| Teraspeed Modeling Services.
| http://www.teraspeedlabs.com
[IBIS Ver]   4.0
[Comment Char] |_char
[File Name]   lpc54113j256uk49.ibs
[File Rev]   3.0
[Source]  Measured and created by Teraspeed Labs
[Date]   10-25-2017
[Notes]   Quality Check of this IBIS model: Model Passes IBIS Check
   Model parses into ICX IS. Simulation done with Hyperlynx.
   1. MIN TYP MAX information is based on Temperature and Voltage
   characteristics only.
   2. Package data measured using Tektronix IConnect Software.
[Disclaimer]
| Use: Teraspeed Labs ("Teraspeed") has
| licensed IBIS models to specific integrated circuit
| suppliers ("IC Vendors") for use and distribution as
| follows: Each IC Vendor may use IBIS Models, and distribute
| them to IC Vendor's customers to use solely for developing
| printed circuit board designs. Users of this model may
| modify the IBIS model to suit its specific applications but
| rights to derivative works and such modifications shall belong
| to Teraspeed. No other distribution of these materials is
| permitted.
| DISCLAIMER OF WARRANTY: UNLESS OTHERWISE AGREED TO IN WRITING
| TERASPEED DISCLAIMS AND USER WAIVES ALL WARRANTIES, EXPRESS
| OR IMPLIED, INCLUDING WARRANTIES OF MERCHANTABILITY AND
| FITNESS FOR A PARTICULAR PURPOSE. IN NO EVENT SHALL
| TERASPEED BE LIABLE FOR ANY DIRECT OR INDIRECT DAMAGES,
| WHETHER IN CONTRACT OR TORT, INCLUDING, WITHOUT LIMITATION,
| LOST PROFITS, BUSINESS INTERRUPTION, OR LOST INFORMATION
| ARISING OUT OF THE USE OF OR THE INABILITY TO USE THE MODEL,
| EVEN IF TERASPEED HAS BEEN ADVISED OF THE POSSIBILITY OF SUCH
| DAMAGES.
[Copyright]
| This file is the legal property of Teraspeed Labs Copyright(c) 2017.
| All other rights are reserved.
[Component] LPC54113J256UK49
[Manufacturer] NXP Semiconductors
| Data Sheet: Rev 1.2, 24 February 2016
[Package]
| 49 Ball BGA / WLCSP49
| variable   typ   min   max
R_pkg  1.000E-02  1.000E-02  1.000E-02
L_pkg  5.322E-10  1.768E-10  7.500E-10
C_pkg  2.129E-14  7.071E-15  3.000E-14
[Pin] signal_name  model_name  R_pin  L_pin C_pin
A1   PIO1_2/ADC0_5   pio1_2   1.000E-02   7.500E-10   3.000E-14
A2   PIO1_4/ADC0_7   pio1_4   1.000E-02   6.374E-10   2.550E-14
A3   VSSA   GND   1.000E-02   7.500E-10   3.000E-14
A4   VDDA   POWER   1.000E-02   7.500E-10   3.000E-14
A5   PIO1_6/ADC0_9   pio1_6   1.000E-02   5.590E-10   2.236E-14
A6   PIO0_0   pio0_0   1.000E-02   6.374E-10   2.550E-14
A7   RTCXIN   rtcxin   1.000E-02   7.500E-10   3.000E-14
B1   PIO1_1/ADC0_4   pio1_1   1.000E-02   6.374E-10   2.550E-14
B2   PIO1_3/ADC0_6   pio1_3   1.000E-02   5.000E-10   2.000E-14
B3   PIO1_5/ADC0_8   pio1_5   1.000E-02   3.953E-10   1.581E-14
B4   VREFP   POWER   1.000E-02   7.500E-10   3.000E-14
B5   PIO1_7/ADC0_10   pio1_7   1.000E-02   3.953E-10   1.581E-14
B6   PIO0_1   pio0_1   1.000E-02   5.000E-10   2.000E-14
B7   RTCXOUT   rtcxout   1.000E-02   6.374E-10   2.550E-14
C1   PIO0_30/ADC0_1   pio0_30   1.000E-02   5.590E-10   2.236E-14
C2   PIO0_31/ADC0_2   pio0_31   1.000E-02   3.953E-10   1.581E-14
C3   PIO1_0/ADC0_3   pio1_0   1.000E-02   2.500E-10   1.000E-14
C4   VDD   POWER   1.000E-02   7.500E-10   3.000E-14
C5   PIO1_8/ADC0_11   pio1_8   1.000E-02   2.500E-10   1.000E-14
C6   PIO0_5   pio0_5   1.000E-02   3.953E-10   1.581E-14
C7   PIO0_4   pio0_4   1.000E-02   5.590E-10   2.236E-14
D1   USB_DM   analog_io   1.000E-02   5.303E-10   2.121E-14
D2   USB_DP   analog_io   1.000E-02   3.536E-10   1.414E-14
D3   PIO0_29/ADC0_0   pio0_29   1.000E-02   1.768E-10   7.071E-15
D4   VSS   GND   1.000E-02   7.500E-10   3.000E-14
D5   PIO0_8   pio0_8   1.000E-02   1.768E-10   7.071E-15
D6   PIO0_7   pio0_7   1.000E-02   3.536E-10   1.414E-14
D7   PIO0_6   pio0_6   1.000E-02   5.303E-10   2.121E-14
E1   PIO0_26   pio0_26   1.000E-02   5.590E-10   2.236E-14
E2   PIO0_25   pio0_25   1.000E-02   3.953E-10   1.581E-14
E3   PIO0_21   pio0_21   1.000E-02   2.500E-10   1.000E-14
E4   VSS   GND   1.000E-02   7.500E-10   3.000E-14
E5   PIO0_11   pio0_11   1.000E-02   2.500E-10   1.000E-14
E6   PIO0_10   pio0_10   1.000E-02   3.953E-10   1.581E-14
E7   PIO0_9   pio0_9   1.000E-02   5.590E-10   2.236E-14
F1   PIO0_24   pio0_24   1.000E-02   6.374E-10   2.550E-14
F2   PIO0_23   pio0_23   1.000E-02   5.000E-10   2.000E-14
F3   PIO0_20/TMS   pio0_20   1.000E-02   3.953E-10   1.581E-14
F4   VDD   POWER   1.000E-02   7.500E-10   3.000E-14
F5   SWCLK/PIO0_16   pio0_16   1.000E-02   3.953E-10   1.581E-14
F6   PIO0_14/TCK   pio0_14   1.000E-02   5.000E-10   2.000E-14
F7   PIO0_12   pio0_12   1.000E-02   6.374E-10   2.550E-14
G1   *RESET   reset   1.000E-02   7.500E-10   3.000E-14
G2   PIO0_22   pio0_22   1.000E-02   6.374E-10   2.550E-14
G3   PIO0_19/TDI   pio0_19   1.000E-02   5.590E-10   2.236E-14
G4   PIO0_18/*TRST   pio0_18   1.000E-02   5.303E-10   2.121E-14
G5   SWDIO/PIO0_17   pio0_17   1.000E-02   5.590E-10   2.236E-14
G6   PIO0_15/TDO   pio0_15   1.000E-02   6.374E-10   2.550E-14
G7   PIO0_13   pio0_13   1.000E-02   7.500E-10   3.000E-14
|**Open drain io pins
[Model Selector]   pio0_23
i2c_norm_hi_1.8v   i2c norm mode,hi drv,Open Drain io,1.8V
i2c_norm_hi_2.5v   i2c norm mode,hi drv,Open Drain io,2.5V
i2c_norm_hi_3.3v   i2c norm mode,hi drv,Open Drain io,3.3V
i2c_norm_lo_1.8v   i2c norm mode,lo drv,Open Drain io,1.8V
i2c_norm_lo_2.5v   i2c norm mode,lo drv,Open Drain io,2.5V
i2c_norm_lo_3.3v   i2c norm mode,lo drv,Open Drain io,3.3V
[Model Selector]   pio0_24
i2c_norm_hi_1.8v   i2c norm mode,hi drv,Open Drain io,1.8V
i2c_norm_hi_2.5v   i2c norm mode,hi drv,Open Drain io,2.5V
i2c_norm_hi_3.3v   i2c norm mode,hi drv,Open Drain io,3.3V
i2c_norm_lo_1.8v   i2c norm mode,lo drv,Open Drain io,1.8V
i2c_norm_lo_2.5v   i2c norm mode,lo drv,Open Drain io,2.5V
i2c_norm_lo_3.3v   i2c norm mode,lo drv,Open Drain io,3.3V
[Model Selector]   pio0_25
i2c_norm_hi_1.8v   i2c norm mode,hi drv,Open Drain io,1.8V
i2c_norm_hi_2.5v   i2c norm mode,hi drv,Open Drain io,2.5V
i2c_norm_hi_3.3v   i2c norm mode,hi drv,Open Drain io,3.3V
i2c_norm_lo_1.8v   i2c norm mode,lo drv,Open Drain io,1.8V
i2c_norm_lo_2.5v   i2c norm mode,lo drv,Open Drain io,2.5V
i2c_norm_lo_3.3v   i2c norm mode,lo drv,Open Drain io,3.3V
[Model Selector]   pio0_26
i2c_norm_hi_1.8v   i2c norm mode,hi drv,Open Drain io,1.8V
i2c_norm_hi_2.5v   i2c norm mode,hi drv,Open Drain io,2.5V
i2c_norm_hi_3.3v   i2c norm mode,hi drv,Open Drain io,3.3V
i2c_norm_lo_1.8v   i2c norm mode,lo drv,Open Drain io,1.8V
i2c_norm_lo_2.5v   i2c norm mode,lo drv,Open Drain io,2.5V
i2c_norm_lo_3.3v   i2c norm mode,lo drv,Open Drain io,3.3V
|**Standard io pins,5Vtol
[Model Selector]   pio0_0
pio_1.8v   GP io,1.8V
pio_2.5v   GP io,2.5V
pio_3.3v   GP io,3.3V
pio_1.8v_pd   GP io,pd,1.8V
pio_2.5v_pd   GP io,pd,2.5V
pio_3.3v_pd   GP io,pd,3.3V
pio_1.8v_pu   GP io,pu,1.8V | Pwrup Default
pio_2.5v_pu   GP io,pu,2.5V | Pwrup Default
pio_3.3v_pu   GP io,pu,3.3V | Pwrup Default
pio_fast_1.8v   GP io,fast slew,1.8V
pio_fast_2.5v   GP io,fast slew,2.5V
pio_fast_3.3v   GP io,fast slew,3.3V
pio_fast_1.8v_pd   GP io,fast slew,pd,1.8V
pio_fast_2.5v_pd   GP io,fast slew,pd,2.5V
pio_fast_3.3v_pd   GP io,fast slew,pd,3.3V
pio_fast_1.8v_pu   GP io,fast slew,pu,1.8V
pio_fast_2.5v_pu   GP io,fast slew,pu,2.5V
pio_fast_3.3v_pu   GP io,fast slew,pu,3.3V
[Model Selector]   pio0_1
pio_1.8v   GP io,1.8V
pio_2.5v   GP io,2.5V
pio_3.3v   GP io,3.3V
pio_1.8v_pd   GP io,pd,1.8V
pio_2.5v_pd   GP io,pd,2.5V
pio_3.3v_pd   GP io,pd,3.3V
pio_1.8v_pu   GP io,pu,1.8V | Pwrup Default
pio_2.5v_pu   GP io,pu,2.5V | Pwrup Default
pio_3.3v_pu   GP io,pu,3.3V | Pwrup Default
pio_fast_1.8v   GP io,fast slew,1.8V
pio_fast_2.5v   GP io,fast slew,2.5V
pio_fast_3.3v   GP io,fast slew,3.3V
pio_fast_1.8v_pd   GP io,fast slew,pd,1.8V
pio_fast_2.5v_pd   GP io,fast slew,pd,2.5V
pio_fast_3.3v_pd   GP io,fast slew,pd,3.3V
pio_fast_1.8v_pu   GP io,fast slew,pu,1.8V
pio_fast_2.5v_pu   GP io,fast slew,pu,2.5V
pio_fast_3.3v_pu   GP io,fast slew,pu,3.3V
[Model Selector]   pio0_4
pio_1.8v   GP io,1.8V
pio_2.5v   GP io,2.5V
pio_3.3v   GP io,3.3V
pio_1.8v_pd   GP io,pd,1.8V
pio_2.5v_pd   GP io,pd,2.5V
pio_3.3v_pd   GP io,pd,3.3V
pio_1.8v_pu   GP io,pu,1.8V | Pwrup Default
pio_2.5v_pu   GP io,pu,2.5V | Pwrup Default
pio_3.3v_pu   GP io,pu,3.3V | Pwrup Default
pio_fast_1.8v   GP io,fast slew,1.8V
pio_fast_2.5v   GP io,fast slew,2.5V
pio_fast_3.3v   GP io,fast slew,3.3V
pio_fast_1.8v_pd   GP io,fast slew,pd,1.8V
pio_fast_2.5v_pd   GP io,fast slew,pd,2.5V
pio_fast_3.3v_pd   GP io,fast slew,pd,3.3V
pio_fast_1.8v_pu   GP io,fast slew,pu,1.8V
pio_fast_2.5v_pu   GP io,fast slew,pu,2.5V
pio_fast_3.3v_pu   GP io,fast slew,pu,3.3V
[Model Selector]   pio0_5
pio_1.8v   GP io,1.8V
pio_2.5v   GP io,2.5V
pio_3.3v   GP io,3.3V
pio_1.8v_pd   GP io,pd,1.8V
pio_2.5v_pd   GP io,pd,2.5V
pio_3.3v_pd   GP io,pd,3.3V
pio_1.8v_pu   GP io,pu,1.8V | Pwrup Default
pio_2.5v_pu   GP io,pu,2.5V | Pwrup Default
pio_3.3v_pu   GP io,pu,3.3V | Pwrup Default
pio_fast_1.8v   GP io,fast slew,1.8V
pio_fast_2.5v   GP io,fast slew,2.5V
pio_fast_3.3v   GP io,fast slew,3.3V
pio_fast_1.8v_pd   GP io,fast slew,pd,1.8V
pio_fast_2.5v_pd   GP io,fast slew,pd,2.5V
pio_fast_3.3v_pd   GP io,fast slew,pd,3.3V
pio_fast_1.8v_pu   GP io,fast slew,pu,1.8V
pio_fast_2.5v_pu   GP io,fast slew,pu,2.5V
pio_fast_3.3v_pu   GP io,fast slew,pu,3.3V
[Model Selector]   pio0_6
pio_1.8v   GP io,1.8V
pio_2.5v   GP io,2.5V
pio_3.3v   GP io,3.3V
pio_1.8v_pd   GP io,pd,1.8V
pio_2.5v_pd   GP io,pd,2.5V
pio_3.3v_pd   GP io,pd,3.3V
pio_1.8v_pu   GP io,pu,1.8V | Pwrup Default
pio_2.5v_pu   GP io,pu,2.5V | Pwrup Default
pio_3.3v_pu   GP io,pu,3.3V | Pwrup Default
pio_fast_1.8v   GP io,fast slew,1.8V
pio_fast_2.5v   GP io,fast slew,2.5V
pio_fast_3.3v   GP io,fast slew,3.3V
pio_fast_1.8v_pd   GP io,fast slew,pd,1.8V
pio_fast_2.5v_pd   GP io,fast slew,pd,2.5V
pio_fast_3.3v_pd   GP io,fast slew,pd,3.3V
pio_fast_1.8v_pu   GP io,fast slew,pu,1.8V
pio_fast_2.5v_pu   GP io,fast slew,pu,2.5V
pio_fast_3.3v_pu   GP io,fast slew,pu,3.3V
[Model Selector]   pio0_7
pio_1.8v   GP io,1.8V
pio_2.5v   GP io,2.5V
pio_3.3v   GP io,3.3V
pio_1.8v_pd   GP io,pd,1.8V
pio_2.5v_pd   GP io,pd,2.5V
pio_3.3v_pd   GP io,pd,3.3V
pio_1.8v_pu   GP io,pu,1.8V | Pwrup Default
pio_2.5v_pu   GP io,pu,2.5V | Pwrup Default
pio_3.3v_pu   GP io,pu,3.3V | Pwrup Default
pio_fast_1.8v   GP io,fast slew,1.8V
pio_fast_2.5v   GP io,fast slew,2.5V
pio_fast_3.3v   GP io,fast slew,3.3V
pio_fast_1.8v_pd   GP io,fast slew,pd,1.8V
pio_fast_2.5v_pd   GP io,fast slew,pd,2.5V
pio_fast_3.3v_pd   GP io,fast slew,pd,3.3V
pio_fast_1.8v_pu   GP io,fast slew,pu,1.8V
pio_fast_2.5v_pu   GP io,fast slew,pu,2.5V
pio_fast_3.3v_pu   GP io,fast slew,pu,3.3V
[Model Selector]   pio0_8
pio_1.8v   GP io,1.8V
pio_2.5v   GP io,2.5V
pio_3.3v   GP io,3.3V
pio_1.8v_pd   GP io,pd,1.8V
pio_2.5v_pd   GP io,pd,2.5V
pio_3.3v_pd   GP io,pd,3.3V
pio_1.8v_pu   GP io,pu,1.8V | Pwrup Default
pio_2.5v_pu   GP io,pu,2.5V | Pwrup Default
pio_3.3v_pu   GP io,pu,3.3V | Pwrup Default
pio_fast_1.8v   GP io,fast slew,1.8V
pio_fast_2.5v   GP io,fast slew,2.5V
pio_fast_3.3v   GP io,fast slew,3.3V
pio_fast_1.8v_pd   GP io,fast slew,pd,1.8V
pio_fast_2.5v_pd   GP io,fast slew,pd,2.5V
pio_fast_3.3v_pd   GP io,fast slew,pd,3.3V
pio_fast_1.8v_pu   GP io,fast slew,pu,1.8V
pio_fast_2.5v_pu   GP io,fast slew,pu,2.5V
pio_fast_3.3v_pu   GP io,fast slew,pu,3.3V
[Model Selector]   pio0_9
pio_1.8v   GP io,1.8V
pio_2.5v   GP io,2.5V
pio_3.3v   GP io,3.3V
pio_1.8v_pd   GP io,pd,1.8V
pio_2.5v_pd   GP io,pd,2.5V
pio_3.3v_pd   GP io,pd,3.3V
pio_1.8v_pu   GP io,pu,1.8V | Pwrup Default
pio_2.5v_pu   GP io,pu,2.5V | Pwrup Default
pio_3.3v_pu   GP io,pu,3.3V | Pwrup Default
pio_fast_1.8v   GP io,fast slew,1.8V
pio_fast_2.5v   GP io,fast slew,2.5V
pio_fast_3.3v   GP io,fast slew,3.3V
pio_fast_1.8v_pd   GP io,fast slew,pd,1.8V
pio_fast_2.5v_pd   GP io,fast slew,pd,2.5V
pio_fast_3.3v_pd   GP io,fast slew,pd,3.3V
pio_fast_1.8v_pu   GP io,fast slew,pu,1.8V
pio_fast_2.5v_pu   GP io,fast slew,pu,2.5V
pio_fast_3.3v_pu   GP io,fast slew,pu,3.3V
[Model Selector]   pio0_10
pio_1.8v   GP io,1.8V
pio_2.5v   GP io,2.5V
pio_3.3v   GP io,3.3V
pio_1.8v_pd   GP io,pd,1.8V
pio_2.5v_pd   GP io,pd,2.5V
pio_3.3v_pd   GP io,pd,3.3V
pio_1.8v_pu   GP io,pu,1.8V | Pwrup Default
pio_2.5v_pu   GP io,pu,2.5V | Pwrup Default
pio_3.3v_pu   GP io,pu,3.3V | Pwrup Default
pio_fast_1.8v   GP io,fast slew,1.8V
pio_fast_2.5v   GP io,fast slew,2.5V
pio_fast_3.3v   GP io,fast slew,3.3V
pio_fast_1.8v_pd   GP io,fast slew,pd,1.8V
pio_fast_2.5v_pd   GP io,fast slew,pd,2.5V
pio_fast_3.3v_pd   GP io,fast slew,pd,3.3V
pio_fast_1.8v_pu   GP io,fast slew,pu,1.8V
pio_fast_2.5v_pu   GP io,fast slew,pu,2.5V
pio_fast_3.3v_pu   GP io,fast slew,pu,3.3V
[Model Selector]   pio0_11
pio_1.8v   GP io,1.8V
pio_2.5v   GP io,2.5V
pio_3.3v   GP io,3.3V
pio_1.8v_pd   GP io,pd,1.8V
pio_2.5v_pd   GP io,pd,2.5V
pio_3.3v_pd   GP io,pd,3.3V
pio_1.8v_pu   GP io,pu,1.8V | Pwrup Default
pio_2.5v_pu   GP io,pu,2.5V | Pwrup Default
pio_3.3v_pu   GP io,pu,3.3V | Pwrup Default
pio_fast_1.8v   GP io,fast slew,1.8V
pio_fast_2.5v   GP io,fast slew,2.5V
pio_fast_3.3v   GP io,fast slew,3.3V
pio_fast_1.8v_pd   GP io,fast slew,pd,1.8V
pio_fast_2.5v_pd   GP io,fast slew,pd,2.5V
pio_fast_3.3v_pd   GP io,fast slew,pd,3.3V
pio_fast_1.8v_pu   GP io,fast slew,pu,1.8V
pio_fast_2.5v_pu   GP io,fast slew,pu,2.5V
pio_fast_3.3v_pu   GP io,fast slew,pu,3.3V
[Model Selector]   pio0_12
pio_1.8v   GP io,1.8V
pio_2.5v   GP io,2.5V
pio_3.3v   GP io,3.3V
pio_1.8v_pd   GP io,pd,1.8V
pio_2.5v_pd   GP io,pd,2.5V
pio_3.3v_pd   GP io,pd,3.3V
pio_1.8v_pu   GP io,pu,1.8V | Pwrup Default
pio_2.5v_pu   GP io,pu,2.5V | Pwrup Default
pio_3.3v_pu   GP io,pu,3.3V | Pwrup Default
pio_fast_1.8v   GP io,fast slew,1.8V
pio_fast_2.5v   GP io,fast slew,2.5V
pio_fast_3.3v   GP io,fast slew,3.3V
pio_fast_1.8v_pd   GP io,fast slew,pd,1.8V
pio_fast_2.5v_pd   GP io,fast slew,pd,2.5V
pio_fast_3.3v_pd   GP io,fast slew,pd,3.3V
pio_fast_1.8v_pu   GP io,fast slew,pu,1.8V
pio_fast_2.5v_pu   GP io,fast slew,pu,2.5V
pio_fast_3.3v_pu   GP io,fast slew,pu,3.3V
[Model Selector]   pio0_13
pio_1.8v   GP io,1.8V
pio_2.5v   GP io,2.5V
pio_3.3v   GP io,3.3V
pio_1.8v_pd   GP io,pd,1.8V
pio_2.5v_pd   GP io,pd,2.5V
pio_3.3v_pd   GP io,pd,3.3V
pio_1.8v_pu   GP io,pu,1.8V | Pwrup Default
pio_2.5v_pu   GP io,pu,2.5V | Pwrup Default
pio_3.3v_pu   GP io,pu,3.3V | Pwrup Default
pio_fast_1.8v   GP io,fast slew,1.8V
pio_fast_2.5v   GP io,fast slew,2.5V
pio_fast_3.3v   GP io,fast slew,3.3V
pio_fast_1.8v_pd   GP io,fast slew,pd,1.8V
pio_fast_2.5v_pd   GP io,fast slew,pd,2.5V
pio_fast_3.3v_pd   GP io,fast slew,pd,3.3V
pio_fast_1.8v_pu   GP io,fast slew,pu,1.8V
pio_fast_2.5v_pu   GP io,fast slew,pu,2.5V
pio_fast_3.3v_pu   GP io,fast slew,pu,3.3V
[Model Selector]   pio0_14
pio_1.8v   GP io,1.8V
pio_2.5v   GP io,2.5V
pio_3.3v   GP io,3.3V
pio_1.8v_pd   GP io,pd,1.8V
pio_2.5v_pd   GP io,pd,2.5V
pio_3.3v_pd   GP io,pd,3.3V
pio_1.8v_pu   GP io,pu,1.8V | Pwrup Default
pio_2.5v_pu   GP io,pu,2.5V | Pwrup Default
pio_3.3v_pu   GP io,pu,3.3V | Pwrup Default
pio_fast_1.8v   GP io,fast slew,1.8V
pio_fast_2.5v   GP io,fast slew,2.5V
pio_fast_3.3v   GP io,fast slew,3.3V
pio_fast_1.8v_pd   GP io,fast slew,pd,1.8V
pio_fast_2.5v_pd   GP io,fast slew,pd,2.5V
pio_fast_3.3v_pd   GP io,fast slew,pd,3.3V
pio_fast_1.8v_pu   GP io,fast slew,pu,1.8V
pio_fast_2.5v_pu   GP io,fast slew,pu,2.5V
pio_fast_3.3v_pu   GP io,fast slew,pu,3.3V
[Model Selector]   pio0_15
pio_1.8v   GP io,1.8V
pio_2.5v   GP io,2.5V
pio_3.3v   GP io,3.3V
pio_1.8v_pd   GP io,pd,1.8V
pio_2.5v_pd   GP io,pd,2.5V
pio_3.3v_pd   GP io,pd,3.3V
pio_1.8v_pu   GP io,pu,1.8V | Pwrup Default
pio_2.5v_pu   GP io,pu,2.5V | Pwrup Default
pio_3.3v_pu   GP io,pu,3.3V | Pwrup Default
pio_fast_1.8v   GP io,fast slew,1.8V
pio_fast_2.5v   GP io,fast slew,2.5V
pio_fast_3.3v   GP io,fast slew,3.3V
pio_fast_1.8v_pd   GP io,fast slew,pd,1.8V
pio_fast_2.5v_pd   GP io,fast slew,pd,2.5V
pio_fast_3.3v_pd   GP io,fast slew,pd,3.3V
pio_fast_1.8v_pu   GP io,fast slew,pu,1.8V
pio_fast_2.5v_pu   GP io,fast slew,pu,2.5V
pio_fast_3.3v_pu   GP io,fast slew,pu,3.3V
[Model Selector]   pio0_16
pio_1.8v   GP io,1.8V
pio_2.5v   GP io,2.5V
pio_3.3v   GP io,3.3V
pio_1.8v_pd   GP io,pd,1.8V
pio_2.5v_pd   GP io,pd,2.5V
pio_3.3v_pd   GP io,pd,3.3V
pio_1.8v_pu   GP io,pu,1.8V | Pwrup Default
pio_2.5v_pu   GP io,pu,2.5V | Pwrup Default
pio_3.3v_pu   GP io,pu,3.3V | Pwrup Default
pio_fast_1.8v   GP io,fast slew,1.8V
pio_fast_2.5v   GP io,fast slew,2.5V
pio_fast_3.3v   GP io,fast slew,3.3V
pio_fast_1.8v_pd   GP io,fast slew,pd,1.8V
pio_fast_2.5v_pd   GP io,fast slew,pd,2.5V
pio_fast_3.3v_pd   GP io,fast slew,pd,3.3V
pio_fast_1.8v_pu   GP io,fast slew,pu,1.8V
pio_fast_2.5v_pu   GP io,fast slew,pu,2.5V
pio_fast_3.3v_pu   GP io,fast slew,pu,3.3V
[Model Selector]   pio0_17
pio_1.8v   GP io,1.8V
pio_2.5v   GP io,2.5V
pio_3.3v   GP io,3.3V
pio_1.8v_pd   GP io,pd,1.8V
pio_2.5v_pd   GP io,pd,2.5V
pio_3.3v_pd   GP io,pd,3.3V
pio_1.8v_pu   GP io,pu,1.8V | Pwrup Default
pio_2.5v_pu   GP io,pu,2.5V | Pwrup Default
pio_3.3v_pu   GP io,pu,3.3V | Pwrup Default
pio_fast_1.8v   GP io,fast slew,1.8V
pio_fast_2.5v   GP io,fast slew,2.5V
pio_fast_3.3v   GP io,fast slew,3.3V
pio_fast_1.8v_pd   GP io,fast slew,pd,1.8V
pio_fast_2.5v_pd   GP io,fast slew,pd,2.5V
pio_fast_3.3v_pd   GP io,fast slew,pd,3.3V
pio_fast_1.8v_pu   GP io,fast slew,pu,1.8V
pio_fast_2.5v_pu   GP io,fast slew,pu,2.5V
pio_fast_3.3v_pu   GP io,fast slew,pu,3.3V
[Model Selector]   pio0_18
pio_1.8v   GP io,1.8V
pio_2.5v   GP io,2.5V
pio_3.3v   GP io,3.3V
pio_1.8v_pd   GP io,pd,1.8V
pio_2.5v_pd   GP io,pd,2.5V
pio_3.3v_pd   GP io,pd,3.3V
pio_1.8v_pu   GP io,pu,1.8V | Pwrup Default
pio_2.5v_pu   GP io,pu,2.5V | Pwrup Default
pio_3.3v_pu   GP io,pu,3.3V | Pwrup Default
pio_fast_1.8v   GP io,fast slew,1.8V
pio_fast_2.5v   GP io,fast slew,2.5V
pio_fast_3.3v   GP io,fast slew,3.3V
pio_fast_1.8v_pd   GP io,fast slew,pd,1.8V
pio_fast_2.5v_pd   GP io,fast slew,pd,2.5V
pio_fast_3.3v_pd   GP io,fast slew,pd,3.3V
pio_fast_1.8v_pu   GP io,fast slew,pu,1.8V
pio_fast_2.5v_pu   GP io,fast slew,pu,2.5V
pio_fast_3.3v_pu   GP io,fast slew,pu,3.3V
[Model Selector]   pio0_19
pio_1.8v   GP io,1.8V
pio_2.5v   GP io,2.5V
pio_3.3v   GP io,3.3V
pio_1.8v_pd   GP io,pd,1.8V
pio_2.5v_pd   GP io,pd,2.5V
pio_3.3v_pd   GP io,pd,3.3V
pio_1.8v_pu   GP io,pu,1.8V | Pwrup Default
pio_2.5v_pu   GP io,pu,2.5V | Pwrup Default
pio_3.3v_pu   GP io,pu,3.3V | Pwrup Default
pio_fast_1.8v   GP io,fast slew,1.8V
pio_fast_2.5v   GP io,fast slew,2.5V
pio_fast_3.3v   GP io,fast slew,3.3V
pio_fast_1.8v_pd   GP io,fast slew,pd,1.8V
pio_fast_2.5v_pd   GP io,fast slew,pd,2.5V
pio_fast_3.3v_pd   GP io,fast slew,pd,3.3V
pio_fast_1.8v_pu   GP io,fast slew,pu,1.8V
pio_fast_2.5v_pu   GP io,fast slew,pu,2.5V
pio_fast_3.3v_pu   GP io,fast slew,pu,3.3V
[Model Selector]   pio0_20
pio_1.8v   GP io,1.8V
pio_2.5v   GP io,2.5V
pio_3.3v   GP io,3.3V
pio_1.8v_pd   GP io,pd,1.8V
pio_2.5v_pd   GP io,pd,2.5V
pio_3.3v_pd   GP io,pd,3.3V
pio_1.8v_pu   GP io,pu,1.8V | Pwrup Default
pio_2.5v_pu   GP io,pu,2.5V | Pwrup Default
pio_3.3v_pu   GP io,pu,3.3V | Pwrup Default
pio_fast_1.8v   GP io,fast slew,1.8V
pio_fast_2.5v   GP io,fast slew,2.5V
pio_fast_3.3v   GP io,fast slew,3.3V
pio_fast_1.8v_pd   GP io,fast slew,pd,1.8V
pio_fast_2.5v_pd   GP io,fast slew,pd,2.5V
pio_fast_3.3v_pd   GP io,fast slew,pd,3.3V
pio_fast_1.8v_pu   GP io,fast slew,pu,1.8V
pio_fast_2.5v_pu   GP io,fast slew,pu,2.5V
pio_fast_3.3v_pu   GP io,fast slew,pu,3.3V
[Model Selector]   pio0_21
pio_1.8v   GP io,1.8V
pio_2.5v   GP io,2.5V
pio_3.3v   GP io,3.3V
pio_1.8v_pd   GP io,pd,1.8V
pio_2.5v_pd   GP io,pd,2.5V
pio_3.3v_pd   GP io,pd,3.3V
pio_1.8v_pu   GP io,pu,1.8V | Pwrup Default
pio_2.5v_pu   GP io,pu,2.5V | Pwrup Default
pio_3.3v_pu   GP io,pu,3.3V | Pwrup Default
pio_fast_1.8v   GP io,fast slew,1.8V
pio_fast_2.5v   GP io,fast slew,2.5V
pio_fast_3.3v   GP io,fast slew,3.3V
pio_fast_1.8v_pd   GP io,fast slew,pd,1.8V
pio_fast_2.5v_pd   GP io,fast slew,pd,2.5V
pio_fast_3.3v_pd   GP io,fast slew,pd,3.3V
pio_fast_1.8v_pu   GP io,fast slew,pu,1.8V
pio_fast_2.5v_pu   GP io,fast slew,pu,2.5V
pio_fast_3.3v_pu   GP io,fast slew,pu,3.3V
[Model Selector]   pio0_22
pio_1.8v   GP io,1.8V
pio_2.5v   GP io,2.5V
pio_3.3v   GP io,3.3V
pio_1.8v_pd   GP io,pd,1.8V
pio_2.5v_pd   GP io,pd,2.5V
pio_3.3v_pd   GP io,pd,3.3V
pio_1.8v_pu   GP io,pu,1.8V | Pwrup Default
pio_2.5v_pu   GP io,pu,2.5V | Pwrup Default
pio_3.3v_pu   GP io,pu,3.3V | Pwrup Default
pio_fast_1.8v   GP io,fast slew,1.8V
pio_fast_2.5v   GP io,fast slew,2.5V
pio_fast_3.3v   GP io,fast slew,3.3V
pio_fast_1.8v_pd   GP io,fast slew,pd,1.8V
pio_fast_2.5v_pd   GP io,fast slew,pd,2.5V
pio_fast_3.3v_pd   GP io,fast slew,pd,3.3V
pio_fast_1.8v_pu   GP io,fast slew,pu,1.8V
pio_fast_2.5v_pu   GP io,fast slew,pu,2.5V
pio_fast_3.3v_pu   GP io,fast slew,pu,3.3V
|**Standard io pins w/analog function
[Model Selector]   pio0_29
pio_1.8v   GP io,1.8V
pio_2.5v   GP io,2.5V
pio_3.3v   GP io,3.3V
pio_1.8v_pd   GP io,pd,1.8V
pio_2.5v_pd   GP io,pd,2.5V
pio_3.3v_pd   GP io,pd,3.3V
pio_1.8v_pu   GP io,pu,1.8V | Pwrup Default
pio_2.5v_pu   GP io,pu,2.5V | Pwrup Default
pio_3.3v_pu   GP io,pu,3.3V | Pwrup Default
pio_fast_1.8v   GP io,fast slew,1.8V
pio_fast_2.5v   GP io,fast slew,2.5V
pio_fast_3.3v   GP io,fast slew,3.3V
pio_fast_1.8v_pd   GP io,fast slew,pd,1.8V
pio_fast_2.5v_pd   GP io,fast slew,pd,2.5V
pio_fast_3.3v_pd   GP io,fast slew,pd,3.3V
pio_fast_1.8v_pu   GP io,fast slew,pu,1.8V
pio_fast_2.5v_pu   GP io,fast slew,pu,2.5V
pio_fast_3.3v_pu   GP io,fast slew,pu,3.3V
analog_1.8v   adc input 1.8v
analog_2.5v   adc input 2.5v
analog_3.3v   adc input 3.3v
[Model Selector]   pio0_30
pio_1.8v   GP io,1.8V
pio_2.5v   GP io,2.5V
pio_3.3v   GP io,3.3V
pio_1.8v_pd   GP io,pd,1.8V
pio_2.5v_pd   GP io,pd,2.5V
pio_3.3v_pd   GP io,pd,3.3V
pio_1.8v_pu   GP io,pu,1.8V | Pwrup Default
pio_2.5v_pu   GP io,pu,2.5V | Pwrup Default
pio_3.3v_pu   GP io,pu,3.3V | Pwrup Default
pio_fast_1.8v   GP io,fast slew,1.8V
pio_fast_2.5v   GP io,fast slew,2.5V
pio_fast_3.3v   GP io,fast slew,3.3V
pio_fast_1.8v_pd   GP io,fast slew,pd,1.8V
pio_fast_2.5v_pd   GP io,fast slew,pd,2.5V
pio_fast_3.3v_pd   GP io,fast slew,pd,3.3V
pio_fast_1.8v_pu   GP io,fast slew,pu,1.8V
pio_fast_2.5v_pu   GP io,fast slew,pu,2.5V
pio_fast_3.3v_pu   GP io,fast slew,pu,3.3V
analog_1.8v   adc input 1.8v
analog_2.5v   adc input 2.5v
analog_3.3v   adc input 3.3v
[Model Selector]   pio0_31
pio_1.8v   GP io,1.8V
pio_2.5v   GP io,2.5V
pio_3.3v   GP io,3.3V
pio_1.8v_pd   GP io,pd,1.8V
pio_2.5v_pd   GP io,pd,2.5V
pio_3.3v_pd   GP io,pd,3.3V
pio_1.8v_pu   GP io,pu,1.8V | Pwrup Default
pio_2.5v_pu   GP io,pu,2.5V | Pwrup Default
pio_3.3v_pu   GP io,pu,3.3V | Pwrup Default
pio_fast_1.8v   GP io,fast slew,1.8V
pio_fast_2.5v   GP io,fast slew,2.5V
pio_fast_3.3v   GP io,fast slew,3.3V
pio_fast_1.8v_pd   GP io,fast slew,pd,1.8V
pio_fast_2.5v_pd   GP io,fast slew,pd,2.5V
pio_fast_3.3v_pd   GP io,fast slew,pd,3.3V
pio_fast_1.8v_pu   GP io,fast slew,pu,1.8V
pio_fast_2.5v_pu   GP io,fast slew,pu,2.5V
pio_fast_3.3v_pu   GP io,fast slew,pu,3.3V
analog_1.8v   adc input 1.8v
analog_2.5v   adc input 2.5v
analog_3.3v   adc input 3.3v
[Model Selector]   pio1_0
pio_1.8v   GP io,1.8V
pio_2.5v   GP io,2.5V
pio_3.3v   GP io,3.3V
pio_1.8v_pd   GP io,pd,1.8V
pio_2.5v_pd   GP io,pd,2.5V
pio_3.3v_pd   GP io,pd,3.3V
pio_1.8v_pu   GP io,pu,1.8V | Pwrup Default
pio_2.5v_pu   GP io,pu,2.5V | Pwrup Default
pio_3.3v_pu   GP io,pu,3.3V | Pwrup Default
pio_fast_1.8v   GP io,fast slew,1.8V
pio_fast_2.5v   GP io,fast slew,2.5V
pio_fast_3.3v   GP io,fast slew,3.3V
pio_fast_1.8v_pd   GP io,fast slew,pd,1.8V
pio_fast_2.5v_pd   GP io,fast slew,pd,2.5V
pio_fast_3.3v_pd   GP io,fast slew,pd,3.3V
pio_fast_1.8v_pu   GP io,fast slew,pu,1.8V
pio_fast_2.5v_pu   GP io,fast slew,pu,2.5V
pio_fast_3.3v_pu   GP io,fast slew,pu,3.3V
analog_1.8v   adc input 1.8v
analog_2.5v   adc input 2.5v
analog_3.3v   adc input 3.3v
[Model Selector]   pio1_1
pio_1.8v   GP io,1.8V
pio_2.5v   GP io,2.5V
pio_3.3v   GP io,3.3V
pio_1.8v_pd   GP io,pd,1.8V
pio_2.5v_pd   GP io,pd,2.5V
pio_3.3v_pd   GP io,pd,3.3V
pio_1.8v_pu   GP io,pu,1.8V | Pwrup Default
pio_2.5v_pu   GP io,pu,2.5V | Pwrup Default
pio_3.3v_pu   GP io,pu,3.3V | Pwrup Default
pio_fast_1.8v   GP io,fast slew,1.8V
pio_fast_2.5v   GP io,fast slew,2.5V
pio_fast_3.3v   GP io,fast slew,3.3V
pio_fast_1.8v_pd   GP io,fast slew,pd,1.8V
pio_fast_2.5v_pd   GP io,fast slew,pd,2.5V
pio_fast_3.3v_pd   GP io,fast slew,pd,3.3V
pio_fast_1.8v_pu   GP io,fast slew,pu,1.8V
pio_fast_2.5v_pu   GP io,fast slew,pu,2.5V
pio_fast_3.3v_pu   GP io,fast slew,pu,3.3V
analog_1.8v   adc input 1.8v
analog_2.5v   adc input 2.5v
analog_3.3v   adc input 3.3v
[Model Selector]   pio1_2
pio_1.8v   GP io,1.8V
pio_2.5v   GP io,2.5V
pio_3.3v   GP io,3.3V
pio_1.8v_pd   GP io,pd,1.8V
pio_2.5v_pd   GP io,pd,2.5V
pio_3.3v_pd   GP io,pd,3.3V
pio_1.8v_pu   GP io,pu,1.8V | Pwrup Default
pio_2.5v_pu   GP io,pu,2.5V | Pwrup Default
pio_3.3v_pu   GP io,pu,3.3V | Pwrup Default
pio_fast_1.8v   GP io,fast slew,1.8V
pio_fast_2.5v   GP io,fast slew,2.5V
pio_fast_3.3v   GP io,fast slew,3.3V
pio_fast_1.8v_pd   GP io,fast slew,pd,1.8V
pio_fast_2.5v_pd   GP io,fast slew,pd,2.5V
pio_fast_3.3v_pd   GP io,fast slew,pd,3.3V
pio_fast_1.8v_pu   GP io,fast slew,pu,1.8V
pio_fast_2.5v_pu   GP io,fast slew,pu,2.5V
pio_fast_3.3v_pu   GP io,fast slew,pu,3.3V
analog_1.8v   adc input 1.8v
analog_2.5v   adc input 2.5v
analog_3.3v   adc input 3.3v
[Model Selector]   pio1_3
pio_1.8v   GP io,1.8V
pio_2.5v   GP io,2.5V
pio_3.3v   GP io,3.3V
pio_1.8v_pd   GP io,pd,1.8V
pio_2.5v_pd   GP io,pd,2.5V
pio_3.3v_pd   GP io,pd,3.3V
pio_1.8v_pu   GP io,pu,1.8V | Pwrup Default
pio_2.5v_pu   GP io,pu,2.5V | Pwrup Default
pio_3.3v_pu   GP io,pu,3.3V | Pwrup Default
pio_fast_1.8v   GP io,fast slew,1.8V
pio_fast_2.5v   GP io,fast slew,2.5V
pio_fast_3.3v   GP io,fast slew,3.3V
pio_fast_1.8v_pd   GP io,fast slew,pd,1.8V
pio_fast_2.5v_pd   GP io,fast slew,pd,2.5V
pio_fast_3.3v_pd   GP io,fast slew,pd,3.3V
pio_fast_1.8v_pu   GP io,fast slew,pu,1.8V
pio_fast_2.5v_pu   GP io,fast slew,pu,2.5V
pio_fast_3.3v_pu   GP io,fast slew,pu,3.3V
analog_1.8v   adc input 1.8v
analog_2.5v   adc input 2.5v
analog_3.3v   adc input 3.3v
[Model Selector]   pio1_4
pio_1.8v   GP io,1.8V
pio_2.5v   GP io,2.5V
pio_3.3v   GP io,3.3V
pio_1.8v_pd   GP io,pd,1.8V
pio_2.5v_pd   GP io,pd,2.5V
pio_3.3v_pd   GP io,pd,3.3V
pio_1.8v_pu   GP io,pu,1.8V | Pwrup Default
pio_2.5v_pu   GP io,pu,2.5V | Pwrup Default
pio_3.3v_pu   GP io,pu,3.3V | Pwrup Default
pio_fast_1.8v   GP io,fast slew,1.8V
pio_fast_2.5v   GP io,fast slew,2.5V
pio_fast_3.3v   GP io,fast slew,3.3V
pio_fast_1.8v_pd   GP io,fast slew,pd,1.8V
pio_fast_2.5v_pd   GP io,fast slew,pd,2.5V
pio_fast_3.3v_pd   GP io,fast slew,pd,3.3V
pio_fast_1.8v_pu   GP io,fast slew,pu,1.8V
pio_fast_2.5v_pu   GP io,fast slew,pu,2.5V
pio_fast_3.3v_pu   GP io,fast slew,pu,3.3V
analog_1.8v   adc input 1.8v
analog_2.5v   adc input 2.5v
analog_3.3v   adc input 3.3v
[Model Selector]   pio1_5
pio_1.8v   GP io,1.8V
pio_2.5v   GP io,2.5V
pio_3.3v   GP io,3.3V
pio_1.8v_pd   GP io,pd,1.8V
pio_2.5v_pd   GP io,pd,2.5V
pio_3.3v_pd   GP io,pd,3.3V
pio_1.8v_pu   GP io,pu,1.8V | Pwrup Default
pio_2.5v_pu   GP io,pu,2.5V | Pwrup Default
pio_3.3v_pu   GP io,pu,3.3V | Pwrup Default
pio_fast_1.8v   GP io,fast slew,1.8V
pio_fast_2.5v   GP io,fast slew,2.5V
pio_fast_3.3v   GP io,fast slew,3.3V
pio_fast_1.8v_pd   GP io,fast slew,pd,1.8V
pio_fast_2.5v_pd   GP io,fast slew,pd,2.5V
pio_fast_3.3v_pd   GP io,fast slew,pd,3.3V
pio_fast_1.8v_pu   GP io,fast slew,pu,1.8V
pio_fast_2.5v_pu   GP io,fast slew,pu,2.5V
pio_fast_3.3v_pu   GP io,fast slew,pu,3.3V
analog_1.8v   adc input 1.8v
analog_2.5v   adc input 2.5v
analog_3.3v   adc input 3.3v
[Model Selector]   pio1_6
pio_1.8v   GP io,1.8V
pio_2.5v   GP io,2.5V
pio_3.3v   GP io,3.3V
pio_1.8v_pd   GP io,pd,1.8V
pio_2.5v_pd   GP io,pd,2.5V
pio_3.3v_pd   GP io,pd,3.3V
pio_1.8v_pu   GP io,pu,1.8V | Pwrup Default
pio_2.5v_pu   GP io,pu,2.5V | Pwrup Default
pio_3.3v_pu   GP io,pu,3.3V | Pwrup Default
pio_fast_1.8v   GP io,fast slew,1.8V
pio_fast_2.5v   GP io,fast slew,2.5V
pio_fast_3.3v   GP io,fast slew,3.3V
pio_fast_1.8v_pd   GP io,fast slew,pd,1.8V
pio_fast_2.5v_pd   GP io,fast slew,pd,2.5V
pio_fast_3.3v_pd   GP io,fast slew,pd,3.3V
pio_fast_1.8v_pu   GP io,fast slew,pu,1.8V
pio_fast_2.5v_pu   GP io,fast slew,pu,2.5V
pio_fast_3.3v_pu   GP io,fast slew,pu,3.3V
analog_1.8v   adc input 1.8v
analog_2.5v   adc input 2.5v
analog_3.3v   adc input 3.3v
[Model Selector]   pio1_7
pio_1.8v   GP io,1.8V
pio_2.5v   GP io,2.5V
pio_3.3v   GP io,3.3V
pio_1.8v_pd   GP io,pd,1.8V
pio_2.5v_pd   GP io,pd,2.5V
pio_3.3v_pd   GP io,pd,3.3V
pio_1.8v_pu   GP io,pu,1.8V | Pwrup Default
pio_2.5v_pu   GP io,pu,2.5V | Pwrup Default
pio_3.3v_pu   GP io,pu,3.3V | Pwrup Default
pio_fast_1.8v   GP io,fast slew,1.8V
pio_fast_2.5v   GP io,fast slew,2.5V
pio_fast_3.3v   GP io,fast slew,3.3V
pio_fast_1.8v_pd   GP io,fast slew,pd,1.8V
pio_fast_2.5v_pd   GP io,fast slew,pd,2.5V
pio_fast_3.3v_pd   GP io,fast slew,pd,3.3V
pio_fast_1.8v_pu   GP io,fast slew,pu,1.8V
pio_fast_2.5v_pu   GP io,fast slew,pu,2.5V
pio_fast_3.3v_pu   GP io,fast slew,pu,3.3V
analog_1.8v   adc input 1.8v
analog_2.5v   adc input 2.5v
analog_3.3v   adc input 3.3v
[Model Selector]   pio1_8
pio_1.8v   GP io,1.8V
pio_2.5v   GP io,2.5V
pio_3.3v   GP io,3.3V
pio_1.8v_pd   GP io,pd,1.8V
pio_2.5v_pd   GP io,pd,2.5V
pio_3.3v_pd   GP io,pd,3.3V
pio_1.8v_pu   GP io,pu,1.8V | Pwrup Default
pio_2.5v_pu   GP io,pu,2.5V | Pwrup Default
pio_3.3v_pu   GP io,pu,3.3V | Pwrup Default
pio_fast_1.8v   GP io,fast slew,1.8V
pio_fast_2.5v   GP io,fast slew,2.5V
pio_fast_3.3v   GP io,fast slew,3.3V
pio_fast_1.8v_pd   GP io,fast slew,pd,1.8V
pio_fast_2.5v_pd   GP io,fast slew,pd,2.5V
pio_fast_3.3v_pd   GP io,fast slew,pd,3.3V
pio_fast_1.8v_pu   GP io,fast slew,pu,1.8V
pio_fast_2.5v_pu   GP io,fast slew,pu,2.5V
pio_fast_3.3v_pu   GP io,fast slew,pu,3.3V
analog_1.8v   adc input 1.8v
analog_2.5v   adc input 2.5v
analog_3.3v   adc input 3.3v
|**Special function pins
[Model Selector]   analog_io
analog_1.8v   analog io,1.8V
analog_2.5v   analog io,2.5V
analog_3.3v   analog io,3.3V
[Model Selector]   reset
reset_1.8v   reset input,1.8V
reset_2.5v   reset input,2.5V
reset_3.3v   reset input,3.3V
[Model Selector]   rtcxin
rtcxin_1.8v   Real Time Clock in,analog pad,1.8V
rtcxin_2.5v   Real Time Clock in,analog pad,2.5V
rtcxin_3.3v   Real Time Clock in,analog pad,3.3V
[Model Selector]   rtcxout
rtcxout_1.8v   Real Time Clock out,analog pad,1.8V
rtcxout_2.5v   Real Time Clock out,analog pad,2.5V
rtcxout_3.3v   Real Time Clock out,analog pad,3.3V
| Models and submodels in the file (36): reset_1.8v (Input), reset_2.5v (Input), reset_3.3v (Input), i2c_norm_hi_1.8v (I/O_open_drain), i2c_norm_lo_1.8v (I/O_open_drain), i2c_norm_hi_2.5v (I/O_open_drain), i2c_norm_lo_2.5v (I/O_open_drain), i2c_norm_hi_3.3v (I/O_open_drain), i2c_norm_lo_3.3v (I/O_open_drain), pio_1.8v (I/O), pio_1.8v_pd (I/O), pio_1.8v_pu (I/O), pio_2.5v (I/O), pio_2.5v_pd (I/O), pio_2.5v_pu (I/O), pio_3.3v (I/O), pio_3.3v_pd (I/O), pio_3.3v_pu (I/O), pio_fast_1.8v (I/O), pio_fast_1.8v_pd (I/O), pio_fast_1.8v_pu (I/O), pio_fast_2.5v (I/O), pio_fast_2.5v_pd (I/O), pio_fast_2.5v_pu (I/O), pio_fast_3.3v (I/O), pio_fast_3.3v_pd (I/O), pio_fast_3.3v_pu (I/O), rtcxout_1.8v (Open_drain), rtcxout_2.5v (Open_drain), rtcxout_3.3v (Open_drain), analog_1.8v (Terminator), analog_2.5v (Terminator), analog_3.3v (Terminator), rtcxin_1.8v (Terminator), rtcxin_2.5v (Terminator), rtcxin_3.3v (Terminator)
